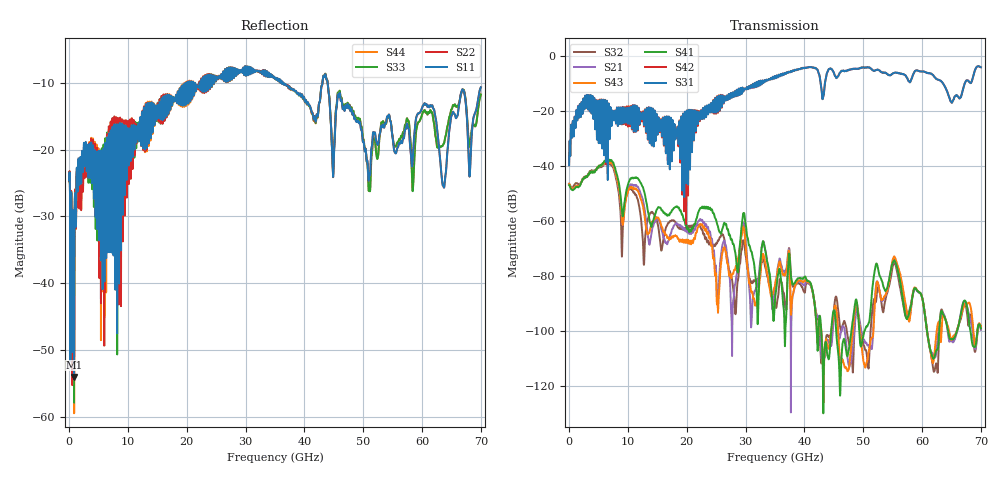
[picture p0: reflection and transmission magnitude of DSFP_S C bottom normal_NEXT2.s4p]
! AWR Design Environment (8415) Wed Jan 09 13:23:47 2019
! Document = 'DSFP_S'
! nPorts: 4, nXvals: 7001
# HZ S DB R 50
!Freq DBS11 AngS11 DBS12 AngS12 DBS13 AngS13 DBS14 AngS14
!	DBS21 AngS21 DBS22 AngS22 DBS23 AngS23 DBS24 AngS24
!	DBS31 AngS31 DBS32 AngS32 DBS33 AngS33 DBS34 AngS34
!	DBS41 AngS41 DBS42 AngS42 DBS43 AngS43 DBS44 AngS44
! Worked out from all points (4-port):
!   7000 points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, 10 MHz to 70 GHz, reference 50 ohm
!   strongest paths, dB at 10 MHz, 17.51 GHz, 35.01 GHz, 52.51 GHz, 70 GHz:
!     S31: -39.7, -27.3, -7.3, -4.9, -4.0
!     S42: -39.3, -27.8, -7.3, -4.9, -4.0
!     S41: -46.9, -55.9, -88.6, -77.1, -99.0
!     S43: -46.4, -65.4, -83.3, -82.6, -98.2
!     S21: -46.4, -62.8, -84.7, -82.7, -99.5
!     S32: -46.7, -59.6, -89.7, -84.1, -98.7
!   lowest |S11| = -54.1 dB at 850 MHz (marker M1), VSWR 1.00, Z = 50.2 + j0.0516 ohm
!   |S11| at or under -10 dB: start of sweep to 20.09 GHz; 36.44 GHz to 43.07 GHz (6.634 GHz wide, 16.7 % of centre); 43.95 GHz to end of sweep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
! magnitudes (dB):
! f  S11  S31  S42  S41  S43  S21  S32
! 10 MHz  -24.6  -39.7  -39.3  -46.9  -46.4  -46.4  -46.7
! 850 MHz  -54.1  -26.2  -26.1  -48.4  -47.9  -48.0  -46.9
! 7.15 GHz  -19.3  -21.3  -21.5  -37.9  -38.7  -38.7  -39.3
! 12.71 GHz  -14.0  -24.3  -25.2  -49.0  -56.4  -54.1  -75.7
! 25.3 GHz  -9.4  -20.2  -20.6  -61.8  -92.8  -88.4  -67.0
! 29.6 GHz  -7.9  -12.9  -12.9  -57.2  -61.9  -60.5  -67.0
! 70 GHz  -10.7  -4.0  -4.0  -99.0  -98.2  -99.5  -98.7
